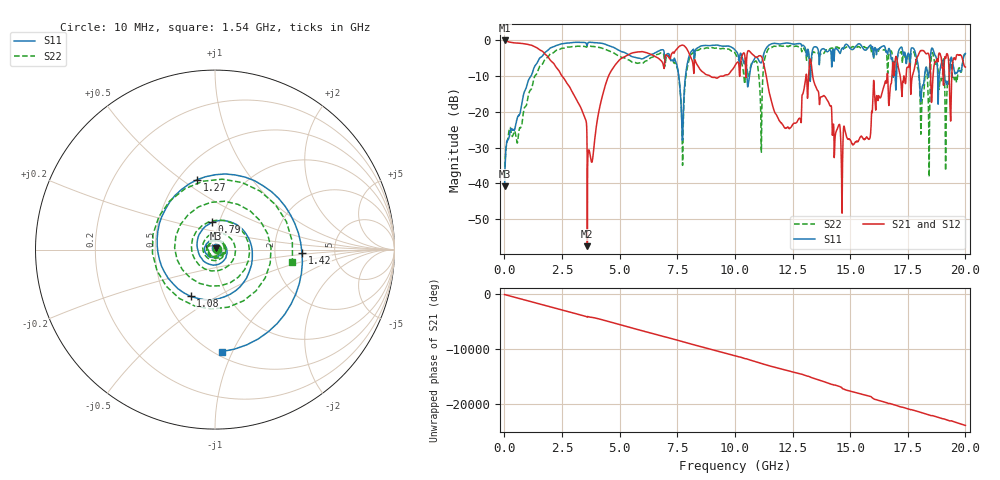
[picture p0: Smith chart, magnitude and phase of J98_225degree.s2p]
!Keysight Technologies,N5222A,MY51421036,A.10.65.16
!Date: Friday, March 31, 2023 15:17:40
!Correction: S11(Full 2 Port(1,2))
!S21(Full 2 Port(1,2))
!S12(Full 2 Port(1,2))
!S22(Full 2 Port(1,2))
!S2P File: Measurements: S11, S21, S12, S22:
# Hz S  dB  R 50
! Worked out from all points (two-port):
!   2000 points, 10 MHz to 20 GHz, reference 50 ohm
!   highest |S21| = -0.01 dB at 10 MHz (marker M1); lowest = -57.5 dB at 3.6 GHz (marker M2)
!   |S21| within 3 dB of the highest: start of sweep to 1.644 GHz; 7.403 GHz to 7.968 GHz (565.6 MHz wide, 7.36 % of centre)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
!   lowest |S11| = -40.7 dB at 10 MHz (marker M3), VSWR 1.02, Z = 50.4 + j0.832 ohm
!   |S11| at or under -10 dB: start of sweep to 1.154 GHz; 7.567 GHz to 7.856 GHz (288.7 MHz wide, 3.74 % of centre); 18 GHz to 18.23 GHz (231.2 MHz wide, 1.28 % of centre)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
!   |S22| runs from -38.3 to -1.4 dB; largest |S21 - S12| = 0.013
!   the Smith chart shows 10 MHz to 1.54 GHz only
!   S11 on the Smith chart (normalised r, x): 10 MHz: 1.01, +0.02; 790 MHz: 0.93, +0.29; 1.08 GHz: 0.67, -0.38; 1.27 GHz: 0.62, +0.57; 1.42 GHz: 2.88, -0.13; 1.54 GHz: 0.54, -0.91
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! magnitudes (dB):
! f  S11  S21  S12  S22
! 10 MHz  -40.7  0.0  0.0  -36.5
! 790 MHz  -16.3  -0.9  -0.9  -21.9
! 1.08 GHz  -10.6  -1.2  -1.2  -14.4
! 1.27 GHz  -7.9  -1.6  -1.6  -11.0
! 1.42 GHz  -6.3  -2.1  -2.1  -9.1
! 1.54 GHz  -4.9  -2.7  -2.7  -7.2
! 3.35 GHz  -0.5  -19.3  -19.3  -1.7
! 3.6 GHz  -1.2  -57.5  -58.5  -1.5
! 4.88 GHz  -2.5  -6.2  -6.2  -4.1
! 6.68 GHz  -3.0  -5.0  -5.0  -3.9
! 7.72 GHz  -28.0  -1.3  -1.3  -29.9
! 8.12 GHz  -3.0  -5.1  -5.1  -3.8
! 10.01 GHz  -2.7  -7.0  -7.0  -3.6
! 11.12 GHz  -6.3  -4.3  -4.3  -19.9
! 12.27 GHz  -0.7  -24.4  -24.3  -1.6
! 13.34 GHz  -3.6  -8.1  -8.1  -4.4
! 14.68 GHz  -2.2  -31.0  -31.1  -2.1
! 16.67 GHz  -2.3  -17.6  -17.6  -4.4
! 17.74 GHz  -2.2  -9.1  -9.1  -3.2
! 18.12 GHz  -13.2  -2.8  -2.8  -17.0
! 18.6 GHz  -2.6  -9.6  -9.6  -3.9
! 20 GHz  -3.6  -7.5  -7.5  -4.3
